[IBIS Ver]   4.2
[File Name]  stm32f2_lqfp64.ibs
[File Rev]   1.0
[Date]   31-Aug-2011
[Source]   STMicroelectronics NV
[Notes]   The I/O models have been made by simulation and qualified
   with recomandation of QualityIBIS flow.
   Some Models, library and pin names may be modified.
   Details of modified names can be found below.
ORIGINAL NAME   ::  MODIFIED NAME   :: COMMENTS(if any)
IO8USB_LSFS_OTG_FT  ::  IO8USB_LSFS_OTG_FT_USB   :: Model in USB mode.
IO8USB_LSFS_OTG_FT  ::  IO8USB_LSFS_OTG_FT_NON_USB_DNV33  :: Model in other than USB mode & pad pin = DNV33
IO8USB_LSFS_OTG_FT  ::  IO8USB_LSFS_OTG_FT_NON_USB_DPV33  :: Model in other than USB mode & pad pin = DPV33
[Disclaimer] These IBIS models are the proprietary information of
   STMicroelectronics and are disclosed to users solely for
   modeling and simulation purposes. No further license is
   implied. All warranties express, implied, or statutory,
   including any implied warranty of fitness for a particular
   purpose or implied warranty against infringement, are
   hereby disclaimed. STMicroelectronics reserves the right
   to change the IBIS models at any time and without notice.
[Copyright]  (c) STMicroelectronics
   All rights reserved. Reproduction in whole or part is prohibited
   without the written consent of the copyright holder.
[Component]  STM32F2_LQFP64
[Manufacturer] STMicroelectronics NV
[Package]
| variable   typ   min   max
R_pkg   0.000mOhm   0.000mOhm   0.000mOhm
L_pkg   0.000nH   0.000nH   0.000nH
C_pkg   0.000pF   0.000pF   0.000pF
[Pin]   signal_name   model_name
|- PE2 IO8PROG2M25M50M100M_ARSUDQ_FT
|- PE3 IO8PROG2M25M50M100M_ARSUDQ_FT
|- PE4 IO8PROG2M25M50M100M_ARSUDQ_FT
|- PE5 IO8PROG2M25M50M100M_ARSUDQ_FT
|- PE6 IO8PROG2M25M50M100M_ARSUDQ_FT
|1 VBAT VDD33IOSWCO_MOSSWI_FT
2 PC13 IO8PROG2M25M50M100M_ARWSUDQ_FT_V33
3 PC14 IO8PROG2M25M50M100M_ARWSUDQ_FT
4 PC15 IO8PROG2M25M50M100M_ARSUDQ_FT
|- VSS_5 VSSIOCO
|- VDD_5 VDD33IOCO
5 PH0 IO8PROG2M25M50M100M_ARSUDQ_FT
6 PH1 IO8PROG2M25M50M100M_ARSUDQ_FT
|7 NRST RESET
8 PC0 IO8PROG2M25M50M100M_AR3WSUDQ_FT
9 PC1 IO8PROG2M25M50M100M_AR3WSUDQ_FT
10 PC2 IO8PROG2M25M50M100M_AR3WSUDQ_FT
11 PC3 IO8PROG2M25M50M100M_AR3WSUDQ_FT
|- VDD_12 VDD33IOCO_VSSIOCO_MOSSWI_FT
|12 VSSA VSSCO
|- VREF+ VDD33CO
|13 VDDA VDD33CO
14 PA0 IO8PROG2M25M50M100M_AR3WSUDQ_FT_V33
15 PA1 IO8PROG2M25M50M100M_AR3WSUDQ_FT
16 PA2 IO8PROG2M25M50M100M_AR3WSUDQ_FT
17 PA3 IO8PROG2M25M50M100M_AR3WSUDQ_FT
|18 VSS_4 VSSIOCO
|19 VDD_4 VDD33IOCO
20 PA4 IO8PROG2M25M50M100M_AR3WSUDQ_FT
21 PA5 IO8PROG2M25M50M100M_AR3WSUDQ_FT
22 PA6 IO8PROG2M25M50M100M_AR3WSUDQ_FT
23 PA7 IO8PROG2M25M50M100M_AR3WSUDQ_FT
24 PC4 IO8PROG2M25M50M100M_AR3WSUDQ_FT
25 PC5 IO8PROG2M25M50M100M_AR3WSUDQ_FT
26 PB0 IO8PROG2M25M50M100M_AR3WSUDQ_FT
27 PB1 IO8PROG2M25M50M100M_AR3WSUDQ_FT
28 PB2 IO8PROG2M25M50M100M_AR3WSUDQ_FT
|- PE7 IO8PROG2M25M50M100M_ARSUDQ_FT
|- PE8 IO8PROG2M25M50M100M_ARSUDQ_FT
|- PE9 IO8PROG2M25M50M100M_ARSUDQ_FT
|- PE10 IO8PROG2M25M50M100M_ARSUDQ_FT
|- PE11 IO8PROG2M25M50M100M_ARSUDQ_FT
|- PE12 IO8PROG2M25M50M100M_ARSUDQ_FT
|- PE13 IO8PROG2M25M50M100M_ARSUDQ_FT
|- PE14 IO8PROG2M25M50M100M_ARSUDQ_FT
|- PE15 IO8PROG2M25M50M100M_ARSUDQ_FT
29 PB10 IO8PROG2M25M50M100M_ARSUDQ_I2CIN_FT
30 PB11 IO8PROG2M25M50M100M_ARSUDQ_I2CIN_FT
|31 VCAP1_0
|32 VDD_1
33 PB12 IO8USB_ID_OTG_FT
34 PB13 IO8USB_VBUS_OTG_FT
|35 PA11 IO8USB_LSFS_OTG_FT_USB
35 PA11 IO8USB_LSFS_OTG_FT_NON_USB_DNV33
|36 PA12 IO8USB_LSFS_OTG_FT_USB
36 PA12 IO8USB_LSFS_OTG_FT_NON_USB_DPV33
|- PD8 IO8PROG2M25M50M100M_ARSUDQ_FT
|- PD9 IO8PROG2M25M50M100M_ARSUDQ_FT
|- PD10 IO8PROG2M25M50M100M_ARSUDQ_FT
|- PD11 IO8PROG2M25M50M100M_ARSUDQ_FT
|- PD12 IO8PROG2M25M50M100M_ARSUDQ_FT
|- PD13 IO8PROG2M25M50M100M_ARSUDQ_FT
|- PD14 IO8PROG2M25M50M100M_ARSUDQ_FT
|- PD15 IO8PROG2M25M50M100M_ARSUDQ_FT
37 PC6 IO8PROG2M25M50M100M_ARSUDQ_FT
38 PC7 IO8PROG2M25M50M100M_ARSUDQ_FT
39 PC8 IO8PROG2M25M50M100M_ARSUDQ_FT
40 PC9 IO8PROG2M25M50M100M_ARSUDQ_I2CIN_FT
41 PA8 IO8PROG2M25M50M100M_ARSUDQ_I2CIN_FT
42 PA9 IO8USB_VBUS_OTG_FT
43 PA10 IO8USB_ID_OTG_FT
44 PA11 IO8USB_LSFS_OTG_FT_USB
|44 PA11 IO8USB_LSFS_OTG_FT_NON_USB_DNV33
45 PA12 IO8USB_LSFS_OTG_FT_USB
|45 PA12 IO8USB_LSFS_OTG_FT_NON_USB_DPV33
46 PA13 IO8PROG2M25M50M100M_ARSUDQ_FT
|47 VCAP2
|- VSS_2
|48 VDD_2
49 PA14 IO8PROG2M25M50M100M_ARSUDQ_FT
50 PA15 IO8PROG2M25M50M100M_AR3WSUDQ_FT
51 PC10 IO8PROG2M25M50M100M_ARSUDQ_FT
52 PC11 IO8PROG2M25M50M100M_ARSUDQ_FT
53 PC12 IO8PROG2M25M50M100M_ARSUDQ_FT
|- PD0 IO8PROG2M25M50M100M_ARSUDQ_FT
|- PD1 IO8PROG2M25M50M100M_ARSUDQ_FT
54 PD2 IO8PROG2M25M50M100M_ARSUDQ_FT
|- PD3 IO8PROG2M25M50M100M_ARSUDQ_FT
|- PD4 IO8PROG2M25M50M100M_ARSUDQ_FT
|- PD5 IO8PROG2M25M50M100M_ARSUDQ_FT
|- PD6 IO8PROG2M25M50M100M_ARSUDQ_FT
|- PD7 IO8PROG2M25M50M100M_ARSUDQ_FT
55 PB3 IO8PROG2M25M50M100M_ARSUDQ_FT
56 PB4 IO8PROG2M25M50M100M_ARSUDQ_FT
57 PB5 IO8PROG2M25M50M100M_AR3WSUDQ_FT
58 PB6 IO8PROG2M25M50M100M_ARSUDQ_I2CIN_FT
59 PB7 IO8PROG2M25M50M100M_ARSUDQ_I2CIN_FT
60 BOOT0 VPP_TEST_HV
61 PB8 IO8PROG2M25M50M100M_ARSUDQ_I2CIN_FT
62 PB9 IO8PROG2M25M50M100M_ARSUDQ_I2CIN_FT
|- PE0 IO8PROG2M25M50M100M_ARSUDQ_FT
|- PE1 IO8PROG2M25M50M100M_ARSUDQ_FT
|- NC
|63 VSS_3
|64 VDD_3  VDD33CO
[Diff Pin]  inv_pin   vdiff tdelay_typ tdelay_min tdelay_max
35 36 200mV 0  0 0
44 45 200mV 0  0 0
[Model Selector] IO8PROG2M25M50M100M_AR3WSUDQ_FT_V33
IO8PROG2M25M50M100M_AR3WSUDQ_DRV_V33_00   DRIVER MODEL  : SPEEDAV33=0 SPEEDBV33=0
IO8PROG2M25M50M100M_AR3WSUDQ_DRV_V33_01   DRIVER MODEL  : SPEEDAV33=0 SPEEDBV33=1
IO8PROG2M25M50M100M_AR3WSUDQ_DRV_V33_10   DRIVER MODEL  : SPEEDAV33=1 SPEEDBV33=0
IO8PROG2M25M50M100M_AR3WSUDQ_DRV_V33_11   DRIVER MODEL  : SPEEDAV33=1 SPEEDBV33=1
IO8PROG2M25M50M100M_AR3WSUDQ_RCV_V33_0   CMOS RECIEVER : ENHYSV33=0  OUTPUT=ZIV33
IO8PROG2M25M50M100M_AR3WSUDQ_RCV_V33_0_T  TTL  RECIEVER : ENHYSV33=0  OUTPUT=ZIV33
IO8PROG2M25M50M100M_AR3WSUDQ_RCV_V33_1   CMOS RECIEVER : ENHYSV33=1  OUTPUT=ZIV33
IO8PROG2M25M50M100M_AR3WSUDQ_RCV_V33_1_T  TTL  RECIEVER : ENHYSV33=1  OUTPUT=ZIV33
[Model Selector] IO8PROG2M25M50M100M_AR3WSUDQ_FT
IO8PROG2M25M50M100M_AR3WSUDQ_FT_DRV_00   DRIVER MODEL  : SPEEDAV12=0 SPEEDBV12=0
IO8PROG2M25M50M100M_AR3WSUDQ_FT_DRV_01   DRIVER MODEL  : SPEEDAV12=0 SPEEDBV12=1
IO8PROG2M25M50M100M_AR3WSUDQ_FT_DRV_10   DRIVER MODEL  : SPEEDAV12=1 SPEEDBV12=0
IO8PROG2M25M50M100M_AR3WSUDQ_FT_DRV_11   DRIVER MODEL  : SPEEDAV12=1 SPEEDBV12=1
IO8PROG2M25M50M100M_AR3WSUDQ_FT_RCV_00   CMOS RECIEVER : ENHYSV12=0  OUTPUT=ZIV12
IO8PROG2M25M50M100M_AR3WSUDQ_FT_RCV_00_T  TTL  RECIEVER : ENHYSV12=0  OUTPUT=ZIV12
IO8PROG2M25M50M100M_AR3WSUDQ_FT_RCV_01   CMOS RECIEVER : ENHYSV12=0  OUTPUT=ZIV33
IO8PROG2M25M50M100M_AR3WSUDQ_FT_RCV_01_T  TTL  RECIEVER : ENHYSV12=0  OUTPUT=ZIV33
IO8PROG2M25M50M100M_AR3WSUDQ_FT_RCV_10   CMOS RECIEVER : ENHYSV12=1  OUTPUT=ZIV12
IO8PROG2M25M50M100M_AR3WSUDQ_FT_RCV_10_T  TTL  RECIEVER : ENHYSV12=1  OUTPUT=ZIV12
IO8PROG2M25M50M100M_AR3WSUDQ_FT_RCV_11   CMOS RECIEVER : ENHYSV12=1  OUTPUT=ZIV33
IO8PROG2M25M50M100M_AR3WSUDQ_FT_RCV_11_T  TTL  RECIEVER : ENHYSV12=1  OUTPUT=ZIV33
[Model Selector] IO8PROG2M25M50M100M_ARSUDQ_FT
IO8PROG2M25M50M100M_ARSUDQ_FT_DRV_00   DRIVER MODEL  : SPEEDAV12=0 SPEEDBV12=0
IO8PROG2M25M50M100M_ARSUDQ_FT_DRV_01   DRIVER MODEL  : SPEEDAV12=0 SPEEDBV12=1
IO8PROG2M25M50M100M_ARSUDQ_FT_DRV_10   DRIVER MODEL  : SPEEDAV12=1 SPEEDBV12=0
IO8PROG2M25M50M100M_ARSUDQ_FT_DRV_11   DRIVER MODEL  : SPEEDAV12=1 SPEEDBV12=1
IO8PROG2M25M50M100M_ARSUDQ_FT_RCV_00   CMOS RECIEVER : ENHYSV12=0  OUTPUT=ZIV12
IO8PROG2M25M50M100M_ARSUDQ_FT_RCV_00_T   TTL  RECIEVER : ENHYSV12=0  OUTPUT=ZIV12
IO8PROG2M25M50M100M_ARSUDQ_FT_RCV_01   CMOS RECIEVER : ENHYSV12=0  OUTPUT=ZIV33
IO8PROG2M25M50M100M_ARSUDQ_FT_RCV_01_T   TTL  RECIEVER : ENHYSV12=0  OUTPUT=ZIV33
IO8PROG2M25M50M100M_ARSUDQ_FT_RCV_10   CMOS RECIEVER : ENHYSV12=1  OUTPUT=ZIV12
IO8PROG2M25M50M100M_ARSUDQ_FT_RCV_10_T   TTL  RECIEVER : ENHYSV12=1  OUTPUT=ZIV12
IO8PROG2M25M50M100M_ARSUDQ_FT_RCV_11   CMOS RECIEVER : ENHYSV12=1  OUTPUT=ZIV33
IO8PROG2M25M50M100M_ARSUDQ_FT_RCV_11_T   TTL  RECIEVER : ENHYSV12=1  OUTPUT=ZIV33
[Model Selector] IO8PROG2M25M50M100M_ARSUDQ_I2CIN_FT
IO8PROG2M25M50M100M_ARSUDQ_I2CIN_DRV_00   DRIVER MODEL  : SPEEDAV12=0 SPEEDBV12=0
IO8PROG2M25M50M100M_ARSUDQ_I2CIN_DRV_01   DRIVER MODEL  : SPEEDAV12=0 SPEEDBV12=1
IO8PROG2M25M50M100M_ARSUDQ_I2CIN_DRV_10   DRIVER MODEL  : SPEEDAV12=1 SPEEDBV12=0
IO8PROG2M25M50M100M_ARSUDQ_I2CIN_DRV_11   DRIVER MODEL  : SPEEDAV12=1 SPEEDBV12=1
IO8PROG2M25M50M100M_I2CIN_RCV_ZII2C_00   CMOS RECIEVER : TESTI2CV12=0  HSFSV12=0
IO8PROG2M25M50M100M_I2CIN_RCV_ZII2C_00_T   TTL  RECIEVER : TESTI2CV12=0  HSFSV12=0
IO8PROG2M25M50M100M_I2CIN_RCV_ZII2C_01   CMOS RECIEVER : TESTI2CV12=0  HSFSV12=1
IO8PROG2M25M50M100M_I2CIN_RCV_ZII2C_01_T   TTL  RECIEVER : TESTI2CV12=0  HSFSV12=1
IO8PROG2M25M50M100M_I2CIN_RCV_ZII2C_10   CMOS RECIEVER : TESTI2CV12=1  HSFSV12=0
IO8PROG2M25M50M100M_I2CIN_RCV_ZII2C_10_T   TTL  RECIEVER : TESTI2CV12=1  HSFSV12=0
IO8PROG2M25M50M100M_I2CIN_RCV_ZII2C_11   CMOS RECIEVER : TESTI2CV12=1  HSFSV12=1
IO8PROG2M25M50M100M_I2CIN_RCV_ZII2C_11_T   TTL  RECIEVER : TESTI2CV12=1  HSFSV12=1
IO8PROG2M25M50M100M_I2CIN_RCV_ZIV12_0   CMOS RECIEVER : ENHYSV12=0  OUTPUT=ZIV12
IO8PROG2M25M50M100M_I2CIN_RCV_ZIV12_0_T   TTL  RECIEVER : ENHYSV12=0  OUTPUT=ZIV12
IO8PROG2M25M50M100M_I2CIN_RCV_ZIV12_1   CMOS RECIEVER : ENHYSV12=1  OUTPUT=ZIV12
IO8PROG2M25M50M100M_I2CIN_RCV_ZIV12_1_T   TTL  RECIEVER : ENHYSV12=1  OUTPUT=ZIV12
IO8PROG2M25M50M100M_I2CIN_RCV_ZIV33_0   CMOS RECIEVER : ENHYSV12=0  OUTPUT=ZIV33
IO8PROG2M25M50M100M_I2CIN_RCV_ZIV33_0_T   TTL  RECIEVER : ENHYSV12=0  OUTPUT=ZIV33
IO8PROG2M25M50M100M_I2CIN_RCV_ZIV33_1   CMOS RECIEVER : ENHYSV12=1  OUTPUT=ZIV33
IO8PROG2M25M50M100M_I2CIN_RCV_ZIV33_1_T   TTL  RECIEVER : ENHYSV12=1  OUTPUT=ZIV33
[Model Selector] IO8PROG2M25M50M100M_ARWSUDQ_FT_V33
IO8PROG2M25M50M100M_ARWSUDQ_DRV_V33_00   DRIVER MODEL  : SPEEDAV33=0 SPEEDBV33=0
IO8PROG2M25M50M100M_ARWSUDQ_DRV_V33_01   DRIVER MODEL  : SPEEDAV33=0 SPEEDBV33=1
IO8PROG2M25M50M100M_ARWSUDQ_DRV_V33_10   DRIVER MODEL  : SPEEDAV33=1 SPEEDBV33=0
IO8PROG2M25M50M100M_ARWSUDQ_DRV_V33_11   DRIVER MODEL  : SPEEDAV33=1 SPEEDBV33=1
IO8PROG2M25M50M100M_ARWSUDQ_RCV_V33_0   CMOS RECIEVER : ENHYSV33=0  OUTPUT=ZIV33
IO8PROG2M25M50M100M_ARWSUDQ_RCV_V33_0_T   TTL  RECIEVER : ENHYSV33=0  OUTPUT=ZIV33
IO8PROG2M25M50M100M_ARWSUDQ_RCV_V33_1   CMOS RECIEVER : ENHYSV33=1  OUTPUT=ZIV33
IO8PROG2M25M50M100M_ARWSUDQ_RCV_V33_1_T   TTL  RECIEVER : ENHYSV33=1  OUTPUT=ZIV33
[Model Selector] IO8PROG2M25M50M100M_ARWSUDQ_FT
IO8PROG2M25M50M100M_ARWSUDQ_FT_DRV_00   DRIVER MODEL  : SPEEDAV12=0 SPEEDBV12=0
IO8PROG2M25M50M100M_ARWSUDQ_FT_DRV_01   DRIVER MODEL  : SPEEDAV12=0 SPEEDBV12=1
IO8PROG2M25M50M100M_ARWSUDQ_FT_DRV_10   DRIVER MODEL  : SPEEDAV12=1 SPEEDBV12=0
IO8PROG2M25M50M100M_ARWSUDQ_FT_DRV_11   DRIVER MODEL  : SPEEDAV12=1 SPEEDBV12=1
IO8PROG2M25M50M100M_ARWSUDQ_FT_RCV_00   CMOS RECIEVER : ENHYSV12=0  OUTPUT=ZIV12
IO8PROG2M25M50M100M_ARWSUDQ_FT_RCV_00_T   TTL  RECIEVER : ENHYSV12=0  OUTPUT=ZIV12
IO8PROG2M25M50M100M_ARWSUDQ_FT_RCV_01   CMOS RECIEVER : ENHYSV12=0  OUTPUT=ZIV33
IO8PROG2M25M50M100M_ARWSUDQ_FT_RCV_01_T   TTL  RECIEVER : ENHYSV12=0  OUTPUT=ZIV33
IO8PROG2M25M50M100M_ARWSUDQ_FT_RCV_10   CMOS RECIEVER : ENHYSV12=1  OUTPUT=ZIV12
IO8PROG2M25M50M100M_ARWSUDQ_FT_RCV_10_T   TTL  RECIEVER : ENHYSV12=1  OUTPUT=ZIV12
IO8PROG2M25M50M100M_ARWSUDQ_FT_RCV_11   CMOS RECIEVER : ENHYSV12=1  OUTPUT=ZIV33
IO8PROG2M25M50M100M_ARWSUDQ_FT_RCV_11_T   TTL  RECIEVER : ENHYSV12=1  OUTPUT=ZIV33
[Model Selector] IO8USB_ID_OTG_FT
IO8USB_ID_OTG_FT_DRV_00   DRIVER MODEL  : SPEEDAV12=0 SPEEDBV12=0
IO8USB_ID_OTG_FT_DRV_01   DRIVER MODEL  : SPEEDAV12=0 SPEEDBV12=1
IO8USB_ID_OTG_FT_DRV_10   DRIVER MODEL  : SPEEDAV12=1 SPEEDBV12=0
IO8USB_ID_OTG_FT_DRV_11   DRIVER MODEL  : SPEEDAV12=1 SPEEDBV12=1
IO8USB_ID_OTG_FT_RCV_00   CMOS RECIEVER : ENHYSV12=0  OUTPUT=ZIV12
IO8USB_ID_OTG_FT_RCV_00_T   TTL  RECIEVER : ENHYSV12=0  OUTPUT=ZIV12
IO8USB_ID_OTG_FT_RCV_01   CMOS RECIEVER : ENHYSV12=0  OUTPUT=ZIV33
IO8USB_ID_OTG_FT_RCV_01_T   TTL  RECIEVER : ENHYSV12=0  OUTPUT=ZIV33
IO8USB_ID_OTG_FT_RCV_10   CMOS RECIEVER : ENHYSV12=1  OUTPUT=ZIV12
IO8USB_ID_OTG_FT_RCV_10_T   TTL  RECIEVER : ENHYSV12=1  OUTPUT=ZIV12
IO8USB_ID_OTG_FT_RCV_11   CMOS RECIEVER : ENHYSV12=1  OUTPUT=ZIV33
IO8USB_ID_OTG_FT_RCV_11_T   TTL  RECIEVER : ENHYSV12=1  OUTPUT=ZIV33
[Model Selector] IO8USB_LSFS_OTG_FT_USB
IO8USB_LSFS_OTG_FT_DRV_USB_0   DRIVER : USBLSFSV12=0 ENUSBV12=0
IO8USB_LSFS_OTG_FT_DRV_USB_1   DRIVER : USBLSFSV12=1 ENUSBV12=0
IO8USB_LSFS_OTG_FT_RCV_USB   USB  RECIEVER : ENHYSV12=1  OUTPUT=USBZIV12
[Model Selector] IO8USB_LSFS_OTG_FT_NON_USB_DNV33
IO8USB_LSFS_OTG_FT_DRV_IO8_DNV33_00   DRIVER : SPEEDAV12=0 SPEEDBV12=0 ENUSBV12=1
IO8USB_LSFS_OTG_FT_DRV_IO8_DNV33_01   DRIVER : SPEEDAV12=0 SPEEDBV12=1 ENUSBV12=1
IO8USB_LSFS_OTG_FT_DRV_IO8_DNV33_10   DRIVER : SPEEDAV12=1 SPEEDBV12=0 ENUSBV12=1
IO8USB_LSFS_OTG_FT_DRV_IO8_DNV33_11   DRIVER : SPEEDAV12=1 SPEEDBV12=1 ENUSBV12=1
IO8USB_LSFS_OTG_FT_RCV_IO8_ZINV12_0   CMOS RECIEVER : ENHYSV12=0  OUTPUT=ZIV12
IO8USB_LSFS_OTG_FT_RCV_IO8_ZINV12_0_T  TTL  RECIEVER : ENHYSV12=0  OUTPUT=ZIV12
IO8USB_LSFS_OTG_FT_RCV_IO8_ZINV12_1   CMOS RECIEVER : ENHYSV12=1  OUTPUT=ZIV12
IO8USB_LSFS_OTG_FT_RCV_IO8_ZINV12_1_T  TTL  RECIEVER : ENHYSV12=1  OUTPUT=ZIV12
IO8USB_LSFS_OTG_FT_RCV_IO8_ZINV33_0   CMOS RECIEVER : ENHYSV12=0  OUTPUT=ZIV33
IO8USB_LSFS_OTG_FT_RCV_IO8_ZINV33_0_T  TTL  RECIEVER : ENHYSV12=0  OUTPUT=ZIV33
IO8USB_LSFS_OTG_FT_RCV_IO8_ZINV33_1   CMOS RECIEVER : ENHYSV12=1  OUTPUT=ZIV33
IO8USB_LSFS_OTG_FT_RCV_IO8_ZINV33_1_T  TTL  RECIEVER : ENHYSV12=1  OUTPUT=ZIV33
[Model Selector] IO8USB_LSFS_OTG_FT_NON_USB_DPV33
IO8USB_LSFS_OTG_FT_DRV_IO8_DPV33_00   DRIVER : SPEEDAV12=0 SPEEDBV12=0 ENUSBV12=1
IO8USB_LSFS_OTG_FT_DRV_IO8_DPV33_01   DRIVER : SPEEDAV12=0 SPEEDBV12=1 ENUSBV12=1
IO8USB_LSFS_OTG_FT_DRV_IO8_DPV33_10   DRIVER : SPEEDAV12=1 SPEEDBV12=0 ENUSBV12=1
IO8USB_LSFS_OTG_FT_DRV_IO8_DPV33_11   DRIVER : SPEEDAV12=1 SPEEDBV12=1 ENUSBV12=1
IO8USB_LSFS_OTG_FT_RCV_IO8_ZIPV12_0   CMOS RECIEVER : ENHYSV12=0  OUTPUT=ZIV12
IO8USB_LSFS_OTG_FT_RCV_IO8_ZIPV12_0_T  TTL  RECIEVER : ENHYSV12=0  OUTPUT=ZIV12
IO8USB_LSFS_OTG_FT_RCV_IO8_ZIPV12_1   CMOS RECIEVER : ENHYSV12=1  OUTPUT=ZIV12
IO8USB_LSFS_OTG_FT_RCV_IO8_ZIPV12_1_T  TTL  RECIEVER : ENHYSV12=1  OUTPUT=ZIV12
IO8USB_LSFS_OTG_FT_RCV_IO8_ZIPV33_0   CMOS RECIEVER : ENHYSV12=0  OUTPUT=ZIV33
IO8USB_LSFS_OTG_FT_RCV_IO8_ZIPV33_0_T  TTL  RECIEVER : ENHYSV12=0  OUTPUT=ZIV33
IO8USB_LSFS_OTG_FT_RCV_IO8_ZIPV33_1   CMOS RECIEVER : ENHYSV12=1  OUTPUT=ZIV33
IO8USB_LSFS_OTG_FT_RCV_IO8_ZIPV33_1_T  TTL  RECIEVER : ENHYSV12=1  OUTPUT=ZIV33
[Model Selector] IO8USB_VBUS_OTG_FT
IO8USB_VBUS_OTG_FT_DRV_00   DRIVER MODEL  : SPEEDAV12=0 SPEEDBV12=0
IO8USB_VBUS_OTG_FT_DRV_01   DRIVER MODEL  : SPEEDAV12=0 SPEEDBV12=1
IO8USB_VBUS_OTG_FT_DRV_10   DRIVER MODEL  : SPEEDAV12=1 SPEEDBV12=0
IO8USB_VBUS_OTG_FT_DRV_11   DRIVER MODEL  : SPEEDAV12=1 SPEEDBV12=1
IO8USB_VBUS_OTG_FT_RCV_00   CMOS RECIEVER : ENHYSV12=0  OUTPUT=ZIV12
IO8USB_VBUS_OTG_FT_RCV_00_T   TTL  RECIEVER : ENHYSV12=0  OUTPUT=ZIV12
IO8USB_VBUS_OTG_FT_RCV_01   CMOS RECIEVER : ENHYSV12=0  OUTPUT=ZIV33
IO8USB_VBUS_OTG_FT_RCV_01_T   TTL  RECIEVER : ENHYSV12=0  OUTPUT=ZIV33
IO8USB_VBUS_OTG_FT_RCV_10   CMOS RECIEVER : ENHYSV12=1  OUTPUT=ZIV12
IO8USB_VBUS_OTG_FT_RCV_10_T   TTL  RECIEVER : ENHYSV12=1  OUTPUT=ZIV12
IO8USB_VBUS_OTG_FT_RCV_11   CMOS RECIEVER : ENHYSV12=1  OUTPUT=ZIV33
IO8USB_VBUS_OTG_FT_RCV_11_T   TTL  RECIEVER : ENHYSV12=1  OUTPUT=ZIV33
[Model Selector] VPP_TEST_HV
VPP_TEST_HV_00   CMOS RECIEVER : ENHYSV12=0  OUTPUT=ZIV12
VPP_TEST_HV_00_T   TTL  RECIEVER : ENHYSV12=0  OUTPUT=ZIV12
VPP_TEST_HV_01   CMOS RECIEVER : ENHYSV12=0  OUTPUT=ZIV33
VPP_TEST_HV_01_T   TTL  RECIEVER : ENHYSV12=0  OUTPUT=ZIV33
VPP_TEST_HV_10   CMOS RECIEVER : ENHYSV12=1  OUTPUT=ZIV12
VPP_TEST_HV_10_T   TTL  RECIEVER : ENHYSV12=1  OUTPUT=ZIV12
VPP_TEST_HV_11   CMOS RECIEVER : ENHYSV12=1  OUTPUT=ZIV33
VPP_TEST_HV_11_T   TTL  RECIEVER : ENHYSV12=1  OUTPUT=ZIV33
| Models and submodels in the file (131): IO8PROG2M25M50M100M_AR3WSUDQ_DRV_V33_00 (3-state), IO8PROG2M25M50M100M_AR3WSUDQ_DRV_V33_01 (3-state), IO8PROG2M25M50M100M_AR3WSUDQ_DRV_V33_10 (3-state), IO8PROG2M25M50M100M_AR3WSUDQ_DRV_V33_11 (3-state), IO8PROG2M25M50M100M_AR3WSUDQ_FT_DRV_00 (3-state), IO8PROG2M25M50M100M_AR3WSUDQ_FT_DRV_01 (3-state), IO8PROG2M25M50M100M_AR3WSUDQ_FT_DRV_10 (3-state), IO8PROG2M25M50M100M_AR3WSUDQ_FT_DRV_11 (3-state), IO8PROG2M25M50M100M_AR3WSUDQ_FT_RCV_00 (Input), IO8PROG2M25M50M100M_AR3WSUDQ_FT_RCV_00_T (Input), IO8PROG2M25M50M100M_AR3WSUDQ_FT_RCV_01 (Input), IO8PROG2M25M50M100M_AR3WSUDQ_FT_RCV_01_T (Input), IO8PROG2M25M50M100M_AR3WSUDQ_FT_RCV_10 (Input), IO8PROG2M25M50M100M_AR3WSUDQ_FT_RCV_10_T (Input), IO8PROG2M25M50M100M_AR3WSUDQ_FT_RCV_11 (Input), IO8PROG2M25M50M100M_AR3WSUDQ_FT_RCV_11_T (Input), IO8PROG2M25M50M100M_AR3WSUDQ_RCV_V33_0 (Input), IO8PROG2M25M50M100M_AR3WSUDQ_RCV_V33_0_T (Input), IO8PROG2M25M50M100M_AR3WSUDQ_RCV_V33_1 (Input), IO8PROG2M25M50M100M_AR3WSUDQ_RCV_V33_1_T (Input), IO8PROG2M25M50M100M_ARSUDQ_FT_DRV_00 (3-state), IO8PROG2M25M50M100M_ARSUDQ_FT_DRV_01 (3-state), IO8PROG2M25M50M100M_ARSUDQ_FT_DRV_10 (3-state), IO8PROG2M25M50M100M_ARSUDQ_FT_DRV_11 (3-state), IO8PROG2M25M50M100M_ARSUDQ_FT_RCV_00 (Input), IO8PROG2M25M50M100M_ARSUDQ_FT_RCV_00_T (Input), IO8PROG2M25M50M100M_ARSUDQ_FT_RCV_01 (Input), IO8PROG2M25M50M100M_ARSUDQ_FT_RCV_01_T (Input), IO8PROG2M25M50M100M_ARSUDQ_FT_RCV_10 (Input), IO8PROG2M25M50M100M_ARSUDQ_FT_RCV_10_T (Input), IO8PROG2M25M50M100M_ARSUDQ_FT_RCV_11 (Input), IO8PROG2M25M50M100M_ARSUDQ_FT_RCV_11_T (Input), IO8PROG2M25M50M100M_ARSUDQ_I2CIN_DRV_00 (3-state), IO8PROG2M25M50M100M_ARSUDQ_I2CIN_DRV_01 (3-state), IO8PROG2M25M50M100M_ARSUDQ_I2CIN_DRV_10 (3-state), IO8PROG2M25M50M100M_ARSUDQ_I2CIN_DRV_11 (3-state), IO8PROG2M25M50M100M_ARWSUDQ_DRV_V33_00 (3-state), IO8PROG2M25M50M100M_ARWSUDQ_DRV_V33_01 (3-state), IO8PROG2M25M50M100M_ARWSUDQ_DRV_V33_10 (3-state), IO8PROG2M25M50M100M_ARWSUDQ_DRV_V33_11 (3-state), IO8PROG2M25M50M100M_ARWSUDQ_FT_DRV_00 (3-state), IO8PROG2M25M50M100M_ARWSUDQ_FT_DRV_01 (3-state), IO8PROG2M25M50M100M_ARWSUDQ_FT_DRV_10 (3-state), IO8PROG2M25M50M100M_ARWSUDQ_FT_DRV_11 (3-state), IO8PROG2M25M50M100M_ARWSUDQ_FT_RCV_00 (Input), IO8PROG2M25M50M100M_ARWSUDQ_FT_RCV_00_T (Input), IO8PROG2M25M50M100M_ARWSUDQ_FT_RCV_01 (Input), IO8PROG2M25M50M100M_ARWSUDQ_FT_RCV_01_T (Input), IO8PROG2M25M50M100M_ARWSUDQ_FT_RCV_10 (Input), IO8PROG2M25M50M100M_ARWSUDQ_FT_RCV_10_T (Input), IO8PROG2M25M50M100M_ARWSUDQ_FT_RCV_11 (Input), IO8PROG2M25M50M100M_ARWSUDQ_FT_RCV_11_T (Input), IO8PROG2M25M50M100M_ARWSUDQ_RCV_V33_0 (Input), IO8PROG2M25M50M100M_ARWSUDQ_RCV_V33_0_T (Input), IO8PROG2M25M50M100M_ARWSUDQ_RCV_V33_1 (Input), IO8PROG2M25M50M100M_ARWSUDQ_RCV_V33_1_T (Input), IO8PROG2M25M50M100M_I2CIN_RCV_ZII2C_00 (Input), IO8PROG2M25M50M100M_I2CIN_RCV_ZII2C_00_T (Input), IO8PROG2M25M50M100M_I2CIN_RCV_ZII2C_01 (Input), IO8PROG2M25M50M100M_I2CIN_RCV_ZII2C_01_T (Input), IO8PROG2M25M50M100M_I2CIN_RCV_ZII2C_10 (Input), IO8PROG2M25M50M100M_I2CIN_RCV_ZII2C_10_T (Input), IO8PROG2M25M50M100M_I2CIN_RCV_ZII2C_11 (Input), IO8PROG2M25M50M100M_I2CIN_RCV_ZII2C_11_T (Input), IO8PROG2M25M50M100M_I2CIN_RCV_ZIV12_0 (Input), IO8PROG2M25M50M100M_I2CIN_RCV_ZIV12_0_T (Input), IO8PROG2M25M50M100M_I2CIN_RCV_ZIV12_1 (Input), IO8PROG2M25M50M100M_I2CIN_RCV_ZIV12_1_T (Input), IO8PROG2M25M50M100M_I2CIN_RCV_ZIV33_0 (Input), IO8PROG2M25M50M100M_I2CIN_RCV_ZIV33_0_T (Input), IO8PROG2M25M50M100M_I2CIN_RCV_ZIV33_1 (Input), IO8PROG2M25M50M100M_I2CIN_RCV_ZIV33_1_T (Input), IO8USB_ID_OTG_FT_DRV_00 (3-state), IO8USB_ID_OTG_FT_DRV_01 (3-state), IO8USB_ID_OTG_FT_DRV_10 (3-state), IO8USB_ID_OTG_FT_DRV_11 (3-state), IO8USB_ID_OTG_FT_RCV_00 (Input), IO8USB_ID_OTG_FT_RCV_00_T (Input), IO8USB_ID_OTG_FT_RCV_01 (Input), IO8USB_ID_OTG_FT_RCV_01_T (Input)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
